| IBIS file k65_180_169mbga_derated.ibs generated by Viper version: 2014.12.11
[IBIS Ver]   4.2
[Comment Char]   |_char
[File Name]   k65_180_169mbga_derated.ibs
[File Rev]   1.0
[Date]   Thu Aug  4 01:23:17 2016
[Source]   FSL Viper 2014.12.11
[Notes]
[Disclaimer] IMPORTANT NOTICE
  This information is provided on an AS IS basis and without warranty.
  IN NO EVENT SHALL Freescale BE LIABLE FOR INCIDENTAL OR CONSEQUENTIAL
  DAMAGES ARISING FROM USE OF THIS INFORMATION. THIS DISCLAIMER OF
  WARRANTY EXTENDS TO THE USER OF THE INFORMATION, AND TO THEIR CUSTOMERS
  OR USERS OF PRODUCTS  AND IS IN LIEU OF ALL WARRANTIES WHETHER EXPRESS,
  IMPLIED, OR STATUTORY, INCLUDING IMPLIED WARRANTIES OF MERCHANTABILITY
  OR FITNESS FOR PARTICULAR PURPOSE.
  Freescale does not represent or warrant that the information furnished
  hereunder is free of infringement of any third party patents,
  copyrights, trade secrets, or other intellectual property rights.
  Freescale does not represent or warrant that the information is free of
  defect, or that it meets any particular standard, requirements or need
  of the user of the infomation or their customers.
  Freescale reserves the right to change the information in this file
  without notice.
   http://www.freescale.com
[Copyright]   (C) Copyright Freescale 2004 - 2016, All Rights Reserved.
|   k65_169mbga
[Component]   k65_169mbga
[Manufacturer]   FREESCALE
[Package]
| variable   typ   min   max
R_pkg   0.11011   0.040884   0.23662
L_pkg   1.846e-9   8.845e-10   4.141e-9
C_pkg   6.441e-13   4.222e-13   1.029e-12
[Pin] signal_name   model_name   R_pin   L_pin   C_pin
A1   PTE0   p_io_fast_84u3v_6m   0.088284  1.724e-9  6.751e-13
A2   PTD14   p_io_fast_84u3v_6m   0.10604   1.885e-9  5.202e-13
A3   PTD15   p_io_fast_84u3v_6m   0.072813  1.429e-9  5.329e-13
A4   PTD2   p_io_fast_84u3v_6m   0.1268   2.628e-9  5.079e-13
A5   PTD1   p_io_fast_84u3v_6m   0.10315   1.867e-9  5.258e-13
A6   PTD0   p_io_fast_84u3v_6m   0.095784  1.805e-9  4.654e-13
A7   PTC25   p_io_fast_84u3v_6m   0.098693  1.943e-9  4.941e-13
A8   PTC10   p_io_fast_84u3v_6m   0.13788   2.629e-9  5.867e-13
A9   PTC11   p_io_fast_84u3v_6m   0.10025   1.725e-9  5.075e-13
A10   PTC6   p_io_fast_84u3v_6m   0.1083   2.023e-9  5.529e-13
A11   PTC5   p_io_fast_84u3v_6m   0.10336   1.774e-9  5.269e-13
A12   PTC3   p_io_fast_hd_84u3v_6m   0.11497   1.867e-9  5.839e-13
A13   PTC2   p_io_fast_84u3v_6m   0.12015   2.043e-9  6.035e-13
B1   PTE1   p_io_fast_84u3v_6m   0.079457  1.578e-9  4.911e-13
B2   PTD12   p_io_fast_84u3v_6m   0.13223   2.267e-9  5.938e-13
B3   PTD13   p_io_fast_84u3v_6m   0.067795  1.317e-9  4.86e-13
B4   PTD3   p_io_fast_84u3v_6m   0.12036   2.299e-9  6.041e-13
B5   PTD4   p_io_fast_hd_84u3v_6m   0.066213  1.288e-9  5.487e-13
B6   PTC29   p_io_fast_84u3v_6m   0.063885  1.243e-9  5.698e-13
B7   PTC24   p_io_fast_84u3v_6m   0.11024   2.085e-9  5.903e-13
B8   PTC13   p_io_fast_84u3v_6m   0.079153  1.498e-9  6.203e-13
B9   PTC12   p_io_fast_84u3v_6m   0.067907  1.279e-9  6.072e-13
B10   PTC7   p_io_fast_84u3v_6m   0.073775  1.391e-9  5.616e-13
B11   PTC4   p_io_fast_hd_84u3v_6m   0.084045  1.472e-9  5.439e-13
B12   PTC1   p_io_fast_84u3v_6m   0.14447   2.465e-9  6.238e-13
B13   PTC0   p_io_fast_84u3v_6m   0.11824   2.236e-9  4.968e-13
C1   PTE2   p_io_fast_84u3v_6m   0.12813   2.253e-9  5.688e-13
C2   PTD11   p_io_fast_84u3v_6m   0.078019  1.437e-9  7.921e-13
C3   VSS   GND   NA   NA   NA
C4   PTD5   p_io_fast_hd_84u3v_6m   0.10225   1.706e-9  7.353e-13
C5   PTD6   p_io_fast_hd_84u3v_6m   0.066879  1.211e-9  5.784e-13
C6   PTC28   p_io_fast_84u3v_6m   0.12133   1.978e-9  6.196e-13
C7   PTC19   p_io_fast_84u3v_6m   0.11526   1.927e-9  6.065e-13
C8   PTC14   p_io_fast_84u3v_6m   0.10524   1.707e-9  7.094e-13
C9   PTC9   p_io_fast_84u3v_6m   0.098189  1.653e-9  6.626e-13
C10   PTC8   p_io_fast_84u3v_6m   0.068755  1.259e-9  5.703e-13
C11   VSS   GND   NA   NA   NA
C12   PTB23   p_io_fast_84u3v_6m   0.13338   2.458e-9  5.75e-13
C13   PTB22   p_io_fast_84u3v_6m   0.10015   2.008e-9  4.7e-13
D1   PTE3   p_io_fast_84u3v_6m   0.12749   2.078e-9  5.609e-13
D2   PTE5   p_io_fast_84u3v_6m   0.06895   1.238e-9  5.415e-13
D3   PTD10   p_io_fast_84u3v_6m   0.088212  1.464e-9  6.75e-13
D4   PTD9   p_io_fast_84u3v_6m   0.086359  1.445e-9  6.351e-13
D5   PTD8   p_io_fast_84u3v_6m   0.090895  1.499e-9  6.563e-13
D6   PTC27   p_io_fast_84u3v_6m   0.10961   1.692e-9  6.521e-13
D7   PTC18   p_io_fast_84u3v_6m   0.098683  1.609e-9  6.313e-13
D8   PTC15   p_io_fast_84u3v_6m   0.11848   1.798e-9  7.788e-13
D9   PTB21   p_io_fast_84u3v_6m   0.13299   2.087e-9  7.054e-13
D10   PTB20   p_io_fast_84u3v_6m   0.12972   2.086e-9  8.17e-13
D11   PTB19   p_io_fast_84u3v_6m   0.097126  1.707e-9  6.323e-13
D12   PTB18   p_io_fast_84u3v_6m   0.13092   2.368e-9  5.747e-13
D13   PTB17   p_io_fast_84u3v_6m   0.098086  1.782e-9  4.671e-13
E1   PTE4   p_io_fast_84u3v_6m   0.12302   2.158e-9  5.725e-13
E2   PTE6   p_io_fast_84u3v_6m   0.083115  1.522e-9  6.058e-13
E3   PTE7   p_io_fast_84u3v_6m   0.068375  1.274e-9  6.195e-13
E4   PTE8   p_io_fast_84u3v_6m   0.14423   2.306e-9  6.975e-13
E5   PTD7   p_io_fast_hd_84u3v_6m   0.12318   1.819e-9  6.974e-13
E6   PTC26   p_io_fast_84u3v_6m   0.13345   1.937e-9  7.248e-13
E7   PTC17   p_io_fast_84u3v_6m   0.15003   2.281e-9  7.375e-13
E8   PTC16   p_io_fast_84u3v_6m   0.11782   1.786e-9  6.875e-13
E9   PTB15   p_io_fast_84u3v_6m   0.16053   2.397e-9  7.727e-13
E10   PTB14   p_io_fast_84u3v_6m   0.10429   1.69e-9   8.031e-13
E11   PTB13   p_io_fast_84u3v_6m   0.080246  1.418e-9  6.367e-13
E12   PTB12   p_io_fast_84u3v_6m   0.10923   1.924e-9  5.831e-13
E13   PTB11   p_io_fast_84u3v_6m   0.11908   2.396e-9  5.122e-13
F1   USB0DM   NC   0.087618  1.523e-9  5.919e-13
F2   VREGIN0   POWER   0.059153  1.207e-9  6.118e-13
F3   PTE9   p_io_fast_84u3v_6m   0.10164   1.691e-9  7.14e-13
F4   PTE10   p_io_fast_84u3v_6m   0.14628   2.299e-9  6.98e-13
F5   PTE17   p_io_fast_84u3v_6m   0.12766   1.884e-9  7.886e-13
F6   PTE18   p_io_fast_84u3v_6m   0.16023   2.252e-9  8.501e-13
F7   PTE19   p_io_fast_84u3v_6m   0.18209   2.453e-9  9.423e-13
F8   PTB16   p_io_fast_84u3v_6m   0.19729   2.706e-9  8.497e-13
F9   PTB9   p_io_fast_84u3v_6m   0.13772   2.065e-9  7.597e-13
F10   PTB8   p_io_fast_84u3v_6m   0.12514   1.937e-9  7.252e-13
F11   PTB7   p_io_fast_84u3v_6m   0.11664   1.876e-9  7.404e-13
F12   PTB6   p_io_fast_84u3v_6m   0.10326   1.765e-9  7.603e-13
F13   PTB5   p_io_fast_84u3v_6m   0.11747   2.2e-9   5.799e-13
G1   USB0DP   NC   0.078806  1.342e-9  5.659e-13
G2   VREGOUT   POWER   0.040884  8.845e-10 6.563e-13
G3   VSS   GND   NA   NA   NA
G4   PTE11   p_io_fast_84u3v_6m   0.12411   1.873e-9  7.486e-13
G5   VDD   POWER   NA   NA   NA
G6   VDD   POWER   NA   NA   NA
G7   VDD   POWER   NA   NA   NA
G8   VSS   GND   NA   NA   NA
G9   PTB10   p_io_fast_84u3v_6m   0.17246   2.448e-9  8.509e-13
G10   PTB3   p_io_fast_84u3v_6m   0.124   1.953e-9  7.197e-13
G11   PTB2   p_io_fast_84u3v_6m   0.091895  1.579e-9  6.23e-13
G12   PTB1   p_io_fast_hd_84u3v_6m   0.07991   1.542e-9  6.198e-13
G13   PTB0   p_io_fast_hd_84u3v_6m   0.11482   1.968e-9  5.687e-13
H1   USB1DM   NC   0.084976  1.423e-9  5.35e-13
H2   VREGIN1   POWER   0.046756  9.19e-10  5.522e-13
H3   PTE16   p_io_fast_84u3v_6m   0.1081   1.64e-9   7.525e-13
H4   PTE12   p_io_fast_84u3v_6m   0.21111   3.055e-9  9.123e-13
H5   VDD   POWER   NA   NA   NA
H6   VDD   POWER   NA   NA   NA
H7   VDD   POWER   NA   NA   NA
H8   VSS   GND   NA   NA   NA
H9   PTB4   p_io_fast_84u3v_6m   0.14694   2.152e-9  7.772e-13
H10   PTA30   p_io_fast_84u3v_6m   0.11935   1.879e-9  7.078e-13
H11   PTA29   p_io_fast_84u3v_6m   0.089266  1.544e-9  6.064e-13
H12   PTA28   p_io_fast_84u3v_6m   0.082375  1.536e-9  6.561e-13
H13   PTA27   p_io_fast_84u3v_6m   0.11821   2.138e-9  5.73e-13
J1   USB1DP   NC   0.078035  1.279e-9  5.12e-13
J2   USB1VBUS   POWER   0.04169   9.428e-10 5.557e-13
J3   VDDA   POWER   0.078547  1.355e-9  6.952e-13
J4   VSSA   GND   0.11415   1.866e-9  1.018e-12
J5   TAMPER7   p_io_84u3v_6m   0.15065   2.101e-9  7.904e-13
J6   TAMPER6   p_io_84u3v_6m   0.11978   1.795e-9  7.074e-13
J8   VSS   GND   NA   NA   NA
J9   PTA31   p_io_fast_84u3v_6m   0.16787   2.471e-9  8.397e-13
J10   PTA26   p_io_fast_84u3v_6m   0.14717   2.202e-9  8.103e-13
J11   PTA25   p_io_fast_84u3v_6m   0.11946   1.896e-9  7.5e-13
J12   PTA17   p_io_fast_84u3v_6m   0.16168   2.379e-9  1.029e-12
J13   PTA16   p_io_fast_84u3v_6m   0.23662   3.403e-9  8.712e-13
K1   VSS   GND   NA   NA   NA
K3   VREFH   POWER   0.067783  1.226e-9  6.945e-13
K4   VREFL   NC   0.087197  1.543e-9  8.516e-13
K5   TAMPER3   p_io_84u3v_6m   0.11831   1.861e-9  7.331e-13
K6   TAMPER5   p_io_84u3v_6m   0.10353   1.664e-9  6.593e-13
K7   PTE25   p_io_fast_84u3v_6m   0.11517   1.736e-9  7.008e-13
K8   PTE26   p_io_fast_84u3v_6m   0.14777   2.232e-9  7.287e-13
K9   PTA8   p_io_fast_84u3v_6m   0.15479   2.376e-9  7.504e-13
K10   PTA9   p_io_fast_84u3v_6m   0.12796   1.979e-9  7.168e-13
K11   PTA24   p_io_fast_84u3v_6m   0.063176  1.218e-9  5.602e-13
K12   PTA15   p_io_fast_84u3v_6m   0.2179   3.067e-9  8.756e-13
K13   PTA14   p_io_fast_84u3v_6m   0.22578   4.141e-9  7.858e-13
L1   ADC1DP1   NC   0.12545   2.064e-9  5.863e-13
L2   ADC0DM0_ADC1DM3   NC   0.13397   2.162e-9  7.063e-13
L3   ADC0SE16_CMP1IN2_ADC0SE21   NC   0.068778  1.345e-9  5.338e-13
L4   TAMPER1   p_io_84u3v_6m   0.071119  1.354e-9  5.4e-13
L5   TAMPER2   p_io_84u3v_6m   0.090422  1.563e-9  6.29e-13
L6   TAMPER4   p_io_84u3v_6m   0.092872  1.561e-9  6.897e-13
L7   PTE24   p_io_fast_84u3v_6m   0.11668   1.851e-9  6.38e-13
L8   PTE27   p_io_fast_84u3v_6m   0.11594   1.795e-9  6.826e-13
L9   PTA4   p_io_flt_84u3v_6m   0.077317  1.383e-9  6.713e-13
L10   PTA7   p_io_fast_84u3v_6m   0.095019  1.552e-9  6.326e-13
L11   PTA13   p_io_fast_84u3v_6m   0.077579  1.377e-9  5.831e-13
L12   PTA12   p_io_fast_84u3v_6m   0.14272   2.283e-9  7.272e-13
L13   RESETB   p_vpp_84u3v_6m   0.065954  1.247e-9  4.222e-13
M1   ADC1DM1   NC   0.13221   2.296e-9  6.099e-13
M2   ADC0DP0_ADC1DP3   NC   0.14768   2.39e-9   7.417e-13
M3   ADC1SE16_CMP2IN2_ADC0SE22   NC   0.086524  1.6e-9   5.521e-13
M4   DAC0OUT_CMP1IN3_ADC0SE23   NC   0.073247  1.424e-9  5.283e-13
M5   TAMPER0_RTCWAKEUP   p_io_84u3v_6m   0.11573   1.979e-9  6.966e-13
M6   VBAT   POWER   0.073811  1.431e-9  7.079e-13
M7   PTE28   p_io_fast_84u3v_6m   0.10601   1.732e-9  6.488e-13
M8   PTA3   p_io_fast_84u3v_6m   0.064647  1.184e-9  4.941e-13
M9   PTA2   p_io_fast_84u3v_6m   0.095232  1.586e-9  6.199e-13
M10   PTA6   p_io_fast_84u3v_6m   0.14861   2.297e-9  7.425e-13
M11   PTA11   p_io_fast_84u3v_6m   0.086832  1.494e-9  6.155e-13
M12   VSS   GND   NA   NA   NA
M13   PTA19   p_io_fast_84u3v_6m   0.073909  1.331e-9  4.261e-13
N1   ADC1DP0_ADC0DP3   NC   0.1536   2.649e-9  6.425e-13
N2   ADC1DM0_ADC0DM3   NC   0.14679   2.503e-9  6.269e-13
N3   VREFOUT_CMP1IN5_CMP0IN5_ADC1SE18   NC   0.10158   1.831e-9  4.94e-13
N4   DAC1OUT_CMP0IN4_CMP2IN3_ADC1SE23   NC   0.10315   1.799e-9  5.263e-13
N5   XTAL32   NC   0.09223   1.746e-9  4.716e-13
N6   EXTAL32   NC   0.1013   1.799e-9  5.202e-13
N7   VSS   GND   NA   NA   NA
N8   PTA0   p_io_fast_84u3v_6m   0.094713  1.668e-9  4.692e-13
N9   PTA1   p_io_fast_84u3v_6m   0.10909   1.758e-9  5.498e-13
N10   PTA5   p_io_fast_84u3v_6m   0.11345   1.735e-9  5.618e-13
N11   PTA10   p_io_fast_84u3v_6m   0.10333   1.754e-9  5.426e-13
N12   VDD   POWER   NA   NA   NA
N13   PTA18   p_io_fast_84u3v_6m   0.092041  1.635e-9  4.626e-13
[Pin Mapping]   pulldown_ref   pullup_ref
A1   NC   NC
A2   NC   NC
A3   NC   NC
A4   NC   NC
A5   NC   NC
A6   NC   NC
A7   NC   NC
A8   NC   NC
A9   NC   NC
A10   NC   NC
A11   NC   NC
A12   NC   NC
A13   NC   NC
B1   NC   NC
B2   NC   NC
B3   NC   NC
B4   NC   NC
B5   NC   NC
B6   NC   NC
B7   NC   NC
B8   NC   NC
B9   NC   NC
B10   NC   NC
B11   NC   NC
B12   NC   NC
B13   NC   NC
C1   NC   NC
C2   NC   NC
C3   VSS   NC
C4   NC   NC
C5   NC   NC
C6   NC   NC
C7   NC   NC
C8   NC   NC
C9   NC   NC
C10   NC   NC
C11   VSS   NC
C12   NC   NC
C13   NC   NC
D1   NC   NC
D2   NC   NC
D3   NC   NC
D4   NC   NC
D5   NC   NC
D6   NC   NC
D7   NC   NC
D8   NC   NC
D9   NC   NC
D10   NC   NC
D11   NC   NC
D12   NC   NC
D13   NC   NC
E1   NC   NC
E2   NC   NC
E3   NC   NC
E4   NC   NC
E5   NC   NC
E6   NC   NC
E7   NC   NC
E8   NC   NC
E9   NC   NC
E10   NC   NC
E11   NC   NC
E12   NC   NC
E13   NC   NC
F1   NC   NC
F2   NC   VREGIN0
F3   NC   NC
F4   NC   NC
F5   NC   NC
F6   NC   NC
F7   NC   NC
F8   NC   NC
F9   NC   NC
F10   NC   NC
F11   NC   NC
F12   NC   NC
F13   NC   NC
G1   NC   NC
G2   NC   VREGOUT
G3   VSS   NC
G4   NC   NC
G5   NC   VDD
G6   NC   VDD
G7   NC   VDD
G8   VSS   NC
G9   NC   NC
G10   NC   NC
G11   NC   NC
G12   NC   NC
G13   NC   NC
H1   NC   NC
H2   NC   VREGIN1
H3   NC   NC
H4   NC   NC
H5   NC   VDD
H6   NC   VDD
H7   NC   VDD
H8   VSS   NC
H9   NC   NC
H10   NC   NC
H11   NC   NC
H12   NC   NC
H13   NC   NC
J1   NC   NC
J2   NC   USB1VBUS
J3   NC   VDDA
J4   VSSA   NC
J5   NC   NC
J6   NC   NC
J8   VSS   NC
J9   NC   NC
J10   NC   NC
J11   NC   NC
J12   NC   NC
J13   NC   NC
K1   VSS   NC
K3   NC   VREFH
K4   NC   NC
K5   NC   NC
K6   NC   NC
K7   NC   NC
K8   NC   NC
K9   NC   NC
K10   NC   NC
K11   NC   NC
K12   NC   NC
K13   NC   NC
L1   NC   NC
L2   NC   NC
L3   NC   NC
L4   NC   NC
L5   NC   NC
L6   NC   NC
L7   NC   NC
L8   NC   NC
L9   NC   NC
L10   NC   NC
L11   NC   NC
L12   NC   NC
L13   NC   NC
M1   NC   NC
M2   NC   NC
M3   NC   NC
M4   NC   NC
M5   NC   NC
M6   NC   VBAT
M7   NC   NC
M8   NC   NC
M9   NC   NC
M10   NC   NC
M11   NC   NC
M12   VSS   NC
M13   NC   NC
N1   NC   NC
N2   NC   NC
N3   NC   NC
N4   NC   NC
N5   NC   NC
N6   NC   NC
N7   VSS   NC
N8   NC   NC
N9   NC   NC
N10   NC   NC
N11   NC   NC
N12   NC   VDD
N13   NC   NC
|*   Model Selector   *
[Model Selector] p_io_84u3v_6m
p_io_84u3v_6m_sre0   io, without slew rate
p_io_84u3v_6m_sre1   io, with slew rate
[Model Selector] p_io_fast_84u3v_6m
p_io_fast_84u3v_6m_sre0   io, without slew rate
p_io_fast_84u3v_6m_sre1   io, with slew rate
[Model Selector] p_io_fast_hd_84u3v_6m
p_io_fast_hd_84u3v_6m_obe1dse0sre0   io 5mA, without slew rate
p_io_fast_hd_84u3v_6m_obe1dse0sre1   io 5mA, with slew rate
p_io_fast_hd_84u3v_6m_obe1dse1sre0   io 20mA, without slew rate
p_io_fast_hd_84u3v_6m_obe1dse1sre1   io 20mA, with slew rate
[Model Selector] p_io_flt_84u3v_6m
p_io_flt_84u3v_6m_sre0   io_flt, without slew rate
p_io_flt_84u3v_6m_sre1   io_flt, with slew rate
| End [Component] k65_169mbga
| Models and submodels in the file (11): p_io_84u3v_6m_sre0 (I/O), p_io_84u3v_6m_sre1 (I/O), p_io_fast_84u3v_6m_sre0 (I/O), p_io_fast_84u3v_6m_sre1 (I/O), p_io_fast_hd_84u3v_6m_obe1dse0sre0 (I/O), p_io_fast_hd_84u3v_6m_obe1dse0sre1 (I/O), p_io_fast_hd_84u3v_6m_obe1dse1sre0 (I/O), p_io_fast_hd_84u3v_6m_obe1dse1sre1 (I/O), p_io_flt_84u3v_6m_sre0 (I/O), p_io_flt_84u3v_6m_sre1 (I/O), p_vpp_84u3v_6m (I/O_open_drain)
